(* Logix 5000 AddOnInstructionDefinition export Banner_WLS_Param_v4; software revision 33.00 *)

TYPE Banner_IOL_Port_v4 :   // UDT that has all of the data items necessary to communicate with a specific Port on a IO-Link Master
STRUCT
   Port_Controlled : INT;   // Each bit represents a port on an IO-Link Master. Set to 1 to tell AOI to control that port.
   Port_Activate : INT;   // Each bit represents a port on an IO-Link Master. When ON that port will process any commands in queue.
   Port_Read : INT;   // Each bit represents a port on an IO-Link Master. Used to determine when device AOI has requested a Read command.
   Port_Write : INT;   // Each bit represents a port on an IO-Link Master. Used to determine when device AOI has requested a Write command.
   Port_RW_Complete : INT;   // Each bit represents a port on an IO-Link Master. Tells device AOI that Read or Write request has been completed.
   Port_Device_Read : INT;
   Data_Transfer : SINT[190];   // Array to transfer data from IO-Master to device AOIs.
END_STRUCT
END_TYPE

TYPE Banner_WLS_CC_v4 :   // Tags to control color for a WLS Pro
STRUCT
   Animation : SINT;   // 0 = Off, 1 = Steady, 2 = Flash, 3 = 2 Color Flash, 4 = 2 Color Shift, 5 = Ends Steady, 6 = Ends Flash, 7 = Scroll, 8 = Center Bounce, 9 = Bounce, 10 = Center Bounce, 11 = Intensity Sweep, 12 = 2 Color Sweep, 13 = Spectrum. WLS15 Only 14 = Level Steady, 15 = Level Flash.
   Color_1 : SINT;   // 0 = Green, 1 = Red, 2 = Orange, 3 = Amber, 4 = Yellow, 5 = Lime Green, 6 = Spring Green, 7 = Cyan, 8 = Sky Blue, 9 = Blue, 10 = Violet, 11 = Magneta, 12 = Rose, 13 = Daylight White, 14 = Custom 1, 15 = Custom 2, 16 = Incandescent, 17 = Warm White, 18 = Flourescent, 19 = Neutral White, 20 = Cool White.
   Color_1_Intensity : SINT;   // 0 = High, 1 = Low, 2 = Medium, 3 = Off, 4 = Custom.
   Speed : SINT;   // 0 = Medium, 1 = Fast, 2 = Slow, 3 = Custom.
   Pulse_Pattern : SINT;   // 0 = Normal, 1 = Strobe, 2 = Three Pulse, 3 = SOS, 4 = Random.
   Color_2 : SINT;   // 0 = Green, 1 = Red, 2 = Orange, 3 = Amber, 4 = Yellow, 5 = Lime Green, 6 = Spring Green, 7 = Cyan, 8 = Sky Blue, 9 = Blue, 10 = Violet, 11 = Magneta, 12 = Rose, 13 = Daylight White, 14 = Custom 1, 15 = Custom 2, 16 = Incandescent, 17 = Warm White, 18 = Flourescent, 19 = Neutral White, 20 = Cool White.
   Color_2_Intensity : SINT;   // 0 = High, 1 = Low, 2 = Medium, 3 = Off, 4 = Custom.
   ScrollBounce : SINT;   // 0 = Solid, 1 = Blended Tail, 2 = Center Blended.
   Percent_Width_C1 : SINT;   // 1 to 100% of Color 1.
   Direction : SINT;   // 0 = Forward, 1 = Backward.
END_STRUCT
END_TYPE

TYPE Banner_WLS_DB_Config_v4 :   // Dim and Blend Mode Config.
STRUCT
   Num_of_Colors : SINT;   // 0 = 1 Color, 1 = 2 Colors, 2 = 3 colors. Number of colors to blend in variable color mode.
   Full_Scale : INT;   // 0 to 100 = Threshold Percent
   Color_1 : SINT;   // 0 = Green, 1 = Red, 2 = Orange, 3 = Amber, 4 = Yellow, 5 = Lime Green, 6 = Spring Green, 7 = Cyan, 8 = Sky Blue, 9 = Blue, 10 = Violet, 11 = Magneta, 12 = Rose, 13 = Daylight White, 14 = Custom 1, 15 = Custom 2, 16 = Incandescent, 17 = Warm White, 18 = Flourescent, 19 = Neutral White, 20 = Cool White.
   Color_1_Intensity : SINT;   // 0 = High, 1 = Low, 2 = Medium, 3 = Off, 4 = Custom
   Color_2 : SINT;   // 0 = Green, 1 = Red, 2 = Orange, 3 = Amber, 4 = Yellow, 5 = Lime Green, 6 = Spring Green, 7 = Cyan, 8 = Sky Blue, 9 = Blue, 10 = Violet, 11 = Magneta, 12 = Rose, 13 = Daylight White, 14 = Custom 1, 15 = Custom 2, 16 = Incandescent, 17 = Warm White, 18 = Flourescent, 19 = Neutral White, 20 = Cool White.
   Color_2_Intensity : SINT;   // 0 = High, 1 = Low, 2 = Medium, 3 = Off, 4 = Custom
   Color_3 : SINT;   // 0 = Green, 1 = Red, 2 = Orange, 3 = Amber, 4 = Yellow, 5 = Lime Green, 6 = Spring Green, 7 = Cyan, 8 = Sky Blue, 9 = Blue, 10 = Violet, 11 = Magneta, 12 = Rose, 13 = Daylight White, 14 = Custom 1, 15 = Custom 2, 16 = Incandescent, 17 = Warm White, 18 = Flourescent, 19 = Neutral White, 20 = Cool White.
   Color_3_Intensity : SINT;   // 0 = High, 1 = Low, 2 = Medium, 3 = Off, 4 = Custom
   Filtering : SINT;   // 0 = None, 1 = Low, 2 = Medium, 3 = High
END_STRUCT
END_TYPE

TYPE Banner_WLS_Gauge_CC_v4 :   // Parameter Data Tags for Gauge mode color control.
STRUCT
   Threshold_Enable : SINT;   // 0 = Disabled, 1 = Enabled.
   Threshold_Value_Percent : SINT;   // 0 to 100 - Threshold %
   Threshold_Comparison : SINT;   // 0 = Less than or equal to, 1 = Greater than or equal to.
   Percent_Width_of_Main_Segment : SINT;   // 0 to 100 = Percent width of color 1
   Main_CC : Banner_WLS_CC_v4;   // Color Control for the Main Lighting.
   Back_CC : Banner_WLS_CC_v4;   // Color Control for the Background Lighting.
END_STRUCT
END_TYPE

TYPE Banner_WLS_Gauge_Config_v4 :   // Tags that control Gauge Mode.
STRUCT
   Full_Scale_Value : INT;   // 0 to 100 = Threshold Percent.
   Filtering : SINT;   // 0 = None, 1 = Low, 2 = Medium, 3 = High
   Hysteresis : SINT;   // 0 = None, 1 = Low, 2 = Medium, 3 = High
   Threshold_Markers_Type : SINT;   // 0 = Off, 1= Non-Dominant, 2= Dominant.
   CC : Banner_WLS_Gauge_CC_v4[3];   // Gauge Color Control tags.
END_STRUCT
END_TYPE

TYPE Banner_WLS_Level_Config_v4 :   // Variables that Control the Level Mode of the WLS Pro.
STRUCT
   Background_Color : SINT;   // 0 = Green, 1 = Red, 2 = Orange, 3 = Amber, 4 = Yellow, 5 = Lime Green, 6 = Spring Green, 7 = Cyan, 8 = Sky Blue, 9 = Blue, 10 = Violet, 11 = Magneta, 12 = Rose, 13 = Daylight White, 14 = Custom 1, 15 = Custom 2, 16 = Incandescent, 17 = Warm White, 18 = Flourescent, 19 = Neutral White, 20 = Cool White.
   Background_Intensity : SINT;   // 0 = High, 1 = Low, 2 = Medium, 3 = Off, 4 = Custom
   Dominance : SINT;   // 0 = Non-Dominant, 1 = Dominant
   SubSegment_Style : SINT;   // 0 = Solid, 1 = Analog
   Filtering : SINT;   // 0 = None, 1 = Low, 2 = Medium, 3 = High
   Hysteresis : SINT;   // 0 = None, 1 = Low, 2 = Medium, 3 = High
   Full_Scale_Value : INT;   // Value that controls what the full scale value is
   Threshold_Marks_Type : SINT;   // WLS15 or WLF only. 0 = Off, 1 = Non-Dominant, 2 = Dominant.
   LB_Config : Banner_WLS_CC_v4;   // Level Base Configuration
   LT_Config : Banner_WLS_LT_v4[5];   // Level Threshold Configuration
END_STRUCT
END_TYPE

TYPE Banner_WLS_LT_v4 :   // Variables to configure the Level Threshold.
STRUCT
   Threshold_Enable : SINT;   // 0 = Threshold Disabled, 1 = Threshold Enabled
   Threshold_Value : SINT;   // 0 to 100 Threshold Percent
   Threshold_Comparison : SINT;   // 0 = Less than or equal to, 1 = Greater than or equal to
   Threshold_Override : SINT;   // 0 = Override not enabled, 1 = Override enabled
   Light_Control : Banner_WLS_CC_v4;   // Color Control
END_STRUCT
END_TYPE

TYPE Banner_WLS_RD_v4 :   // UDT that stores the Read Data for a WLS Pro.
STRUCT
   Master_Cycle_Time : INT;
   Min_Cycle_Time : INT;
   M_Sequence_Capability : INT;
   IO_Link_Version_ID : INT;
   Process_Data_Input_Length : INT;
   Process_Data_Output_Length : INT;
   Combined_Vendor_ID : DINT;   // IO-Link Vendor ID
   Vendor_ID1 : INT;
   Vendor_ID2 : INT;
   Combined_Device_ID : DINT;   // IO-Link Device ID
   Device_ID1 : INT;
   Device_ID2 : INT;
   Device_ID3 : INT;
   Serial_Number : STRING;
END_STRUCT
END_TYPE

TYPE Banner_WLS_Seg_Config_v4 :   // UDT for segment setup in index 66 of the parameter data.
STRUCT
   Basic_Color : SINT;   // 0 = Green, 1 = Red, 2 = Orange, 3 = Amber, 4 = Yellow, 5 = Lime Green, 6 = Spring Green, 7 = Cyan, 8 = Sky Blue, 9 = Blue, 10 = Violet, 11 = Magneta, 12 = Rose, 13 = Daylight White, 14 = Custom 1, 15 = Custom 2, 16 = Incandescent, 17 = Warm White, 18 = Flourescent, 19 = Neutral White, 20 = Cool White.
   Basic_Flash_Rate : SINT;   // 0 = Medium, 1 = Fast, 2 = Slow, 3 = Custom.
   CC : Banner_WLS_CC_v4;   // Color Control
   Manual_Segment_Offset : SINT;   // 0 to 64 = Manual Offset in LEDs.
   Manual_Segment_Width : SINT;   // 0 to 64 = Manual width in LEDs.
END_STRUCT
END_TYPE

TYPE Banner_WLS_v4 :   // All of the parameters for a WLS Pro.
STRUCT
   Initial_Global_Read : BOOL;   // Determines if all of the IO-Link data has been read into the PLC yet
   Command : INT;   // Value placed in here will activate a read or write to a specifc IO-Link Index
   Read : Banner_WLS_RD_v4;   // Read Only Data
   Write : Banner_WLS_WD_v4;   // Write Data
   Archive : Banner_WLS_WD_v4;   // Archive of the Write Data
   Reset : BOOL;   // Resets AOI. This will force a complete parameter read of the sensor.
END_STRUCT
END_TYPE

TYPE Banner_WLS_WD_v4 :   // UDT that stores the Write Data for a WLS Pro.
STRUCT
   System_Command : INT;   // See IODD file for list of commands that can be activated via the System Command interface
   Parameter_Access_Lock : SINT;   // Write access to all parameters is prohibited while value is 1. Only this parameter can be adjusted when value is 1.
   Data_Storage_Lock : SINT;   // Automatic data storage is disabled when this value is equal to 1. Read access is not affected.
   Local_Parameterization_Lock : SINT;   // Parameterization via local control elements on device is disabled.
   Local_User_Interface_Lock : SINT;   // Operation of local user interface is disabled.
   Operating_Mode_Selection : SINT;   // 0 = Segment, 1 = Run, 2 = Level, 3 = Dim & Blend, 4 = Gauge, 5 = LED
   Segment_Mode : SINT;   // 0 = Manual Segment Config. 1 trough 10 = Number of segments in Segment Mode.
   BackGround_Color : SINT;   // 0 = Green, 1 = Red, 2 = Orange, 3 = Amber, 4 = Yellow, 5 = Lime Green, 6 = Spring Green, 7 = Cyan, 8 = Sky Blue, 9 = Blue, 10 = Violet, 11 = Magneta, 12 = Rose, 13 = Daylight White, 14 = Custom 1, 15 = Custom 2, 16 = Incandescent, 17 = Warm White, 18 = Flourescent, 19 = Neutral White, 20 = Cool White.
   Background_Intensity : SINT;   // 0 = High, 1 = Low, 2 = Medium, 3 = Off, 4 = Custom
   Animation_Sync : SINT;   // 0 = Instant Update, 1 = Synchronized Update.
   SM_Config : Banner_WLS_Seg_Config_v4[11];   // Segement Mode Configuration
   LM_Config : Banner_WLS_Level_Config_v4;   // Level Mode Configuration
   Custom_Color_1_R : INT;   // 0 to 255 for Red Custom Color 1.
   Custom_Color_1_G : INT;   // 0 to 255 for Green Custom Color 1.
   Custom_Color_1_B : INT;   // 0 to 255 for Blue Custom Color 1.
   Custom_Color_2_R : INT;   // 0 to 255 for Red Custom Color 2.
   Custom_Color_2_G : INT;   // 0 to 255 for Green Custom Color 2.
   Custom_Color_2_B : INT;   // 0 to 255 for Blue Custom Color 2.
   LED_Mode_Intensity : SINT;   // 0 = High, 1 = Low, 2 = Medium, 3 = Off, 4 = Custom
   Orientation : SINT;   // 0 = Standard, 1 = Upside Down
   Custom_Intensity : SINT;   // 0 to 100 %
   Custom_Frequency : SINT;   // 0 to 255Hz
   DB_Config : Banner_WLS_DB_Config_v4;   // Dim and Blend Configuration
   G_Config : Banner_WLS_Gauge_Config_v4;   // Gauge Configuration
   Number_of_LEDs : INT;
END_STRUCT
END_TYPE

ADD_ON_INSTRUCTION Banner_WLS_Param_v4   (* revision 4.2, vendor Banner Engineering *)
// AOI to read and write parameter data to an IO-Link WLS Pro.
// Revision note:
// Updated for WLF lights.
VAR_IN_OUT
   WLS : Banner_WLS_v4; {required}
   Port_Data : Banner_IOL_Port_v4; {required}
END_VAR
VAR_INPUT
   Port : INT; {required}   // Port Number that device is plugged into.
   Type : SINT; {required}   // 0 = WLS27, 1 = WLS15, 2 = WLF
END_VAR
VAR
   Local_Control : DINT; {access None}
   Global_Read_Command_Value : INT; {access None}
   Global_Write_Command_Value : INT; {access None}
   Command_Being_Processed : BOOL; {access None}
   Update_Archive : BOOL; {access None}
   Index_Write_Inprocess : DINT; {access None}
   Index_Write_Control : DINT; {access None}
   Inprocess_Index : DINT; {access None}
   IndexR : DINT; {access None}   // Index keeping track of Reads in an array.
   S_Index : DINT; {access None}
   IndexW : DINT; {access None}   // Index keeping track of Writes in an array.
   SW_Index : DINT; {access None}
   Index_Segment_Read : DINT; {access None}
   LT_Index : DINT; {access None}
   IndexW2 : DINT; {access None}
   LTW_Index : DINT; {access None}
   G_Index : DINT; {access None}
   IndexW3 : DINT; {access None}
   GW_Index : DINT; {access None}
END_VAR

ROUTINE Logic   (* ladder *)
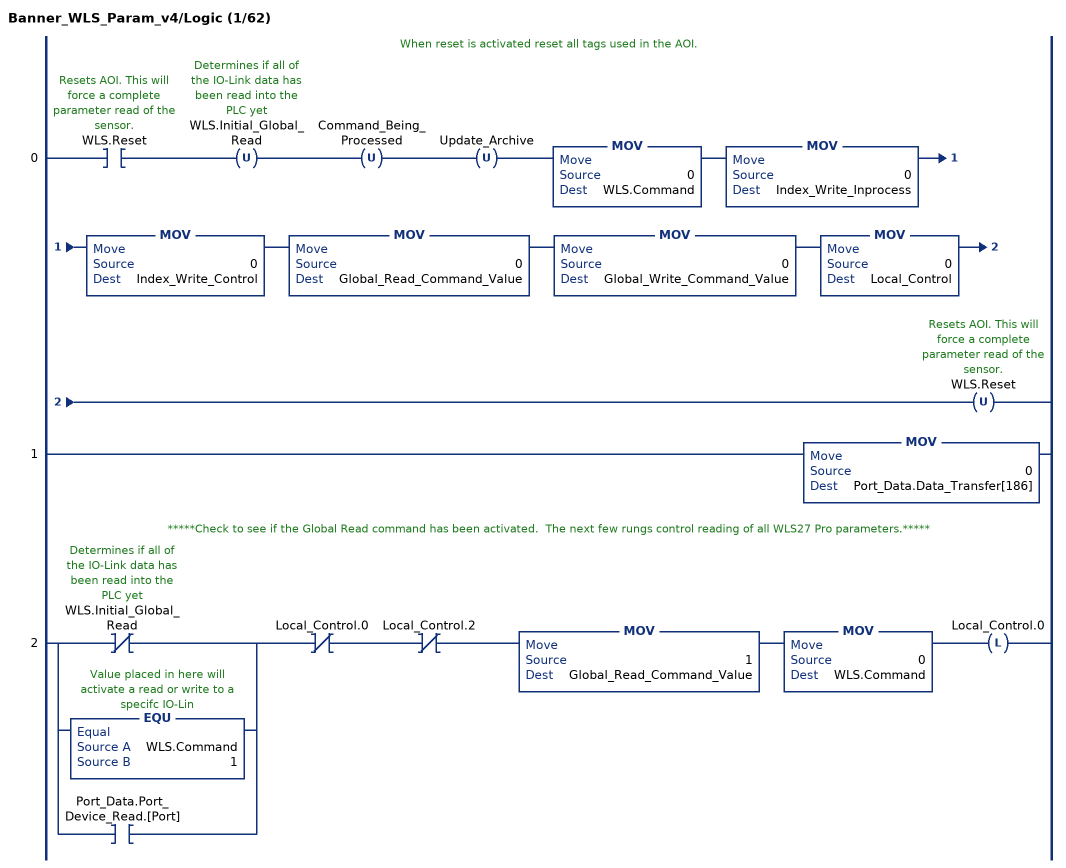
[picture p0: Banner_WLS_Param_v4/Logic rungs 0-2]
   // When reset is activated reset all tags used in the AOI.
   0: XIC(WLS.Reset)OTU(WLS.Initial_Global_Read)OTU(Command_Being_Processed)OTU(Update_Archive)MOV(0,WLS.Command)MOV(0,Index_Write_Inprocess)MOV(0,Index_Write_Control)MOV(0,Global_Read_Command_Value)MOV(0,Global_Write_Command_Value)MOV(0,Local_Control)OTU(WLS.Reset);
   1: MOV(0,Port_Data.Data_Transfer[186]);
   // *****Check to see if the Global Read command has been activated.  The next few rungs control reading of all WLS27 Pro parameters.*****
   2: [XIO(WLS.Initial_Global_Read) ,EQU(WLS.Command,1) ,XIC(Port_Data.Port_Device_Read.[Port]) ]XIO(Local_Control.0)XIO(Local_Control.2)MOV(1,Global_Read_Command_Value)MOV(0,WLS.Command)OTL(Local_Control.0);
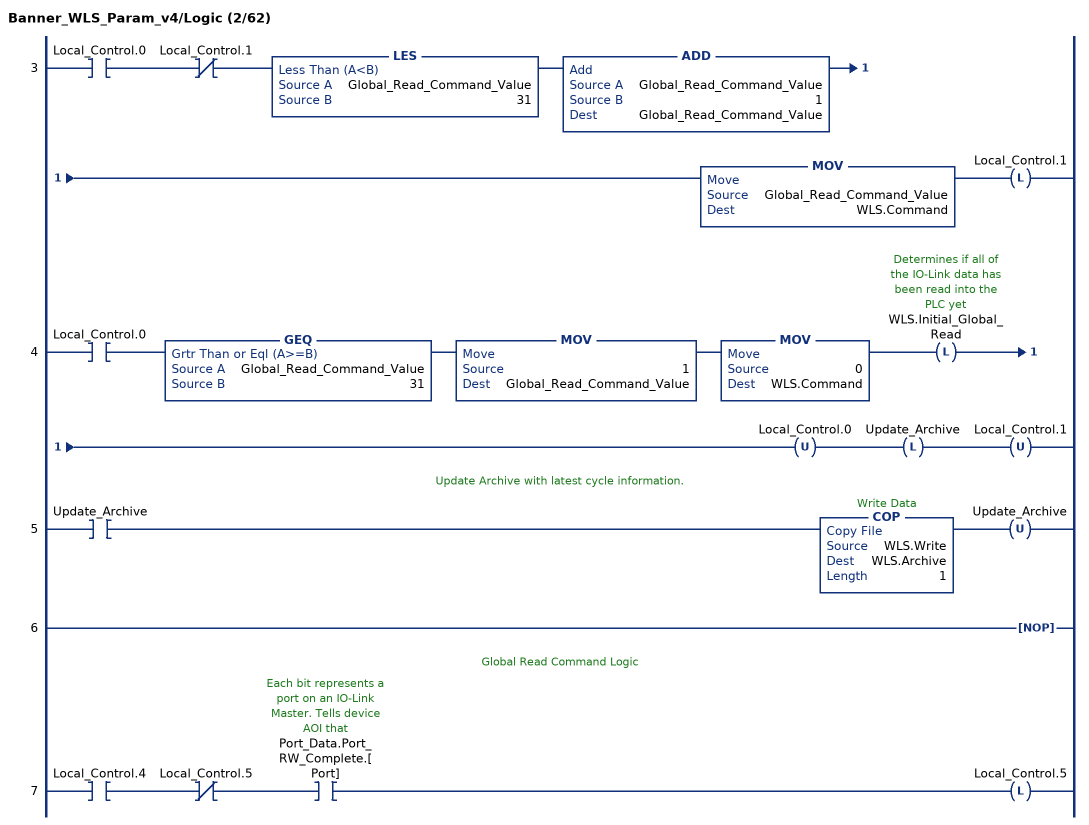
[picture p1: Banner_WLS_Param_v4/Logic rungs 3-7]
   3: XIC(Local_Control.0)XIO(Local_Control.1)LES(Global_Read_Command_Value,31)ADD(Global_Read_Command_Value,1,Global_Read_Command_Value)MOV(Global_Read_Command_Value,WLS.Command)OTL(Local_Control.1);
   4: XIC(Local_Control.0)GEQ(Global_Read_Command_Value,31)MOV(1,Global_Read_Command_Value)MOV(0,WLS.Command)OTL(WLS.Initial_Global_Read)OTU(Local_Control.0)OTL(Update_Archive)OTU(Local_Control.1);
   // Update Archive with latest cycle information.
   5: XIC(Update_Archive)COP(WLS.Write,WLS.Archive,1)OTU(Update_Archive);
   6: NOP();
   // Global Read Command Logic
   7: XIC(Local_Control.4)XIO(Local_Control.5)XIC(Port_Data.Port_RW_Complete.[Port])OTL(Local_Control.5);
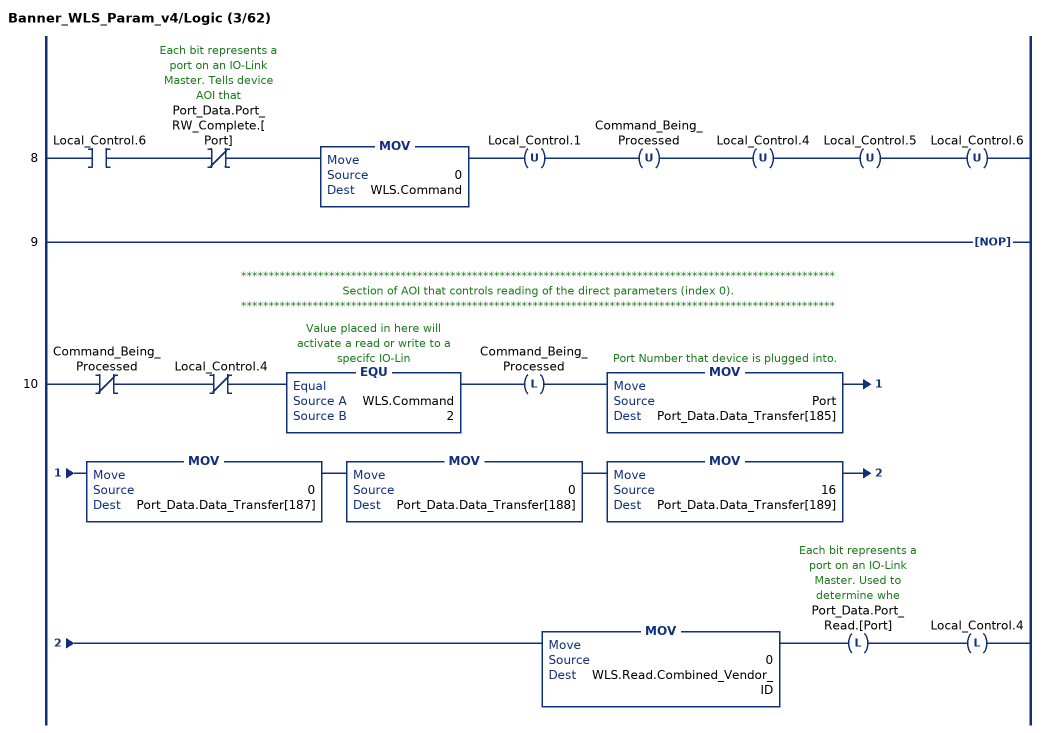
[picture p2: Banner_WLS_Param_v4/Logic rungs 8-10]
   8: XIC(Local_Control.6)XIO(Port_Data.Port_RW_Complete.[Port])MOV(0,WLS.Command)OTU(Local_Control.1)OTU(Command_Being_Processed)OTU(Local_Control.4)OTU(Local_Control.5)OTU(Local_Control.6);
   9: NOP();
   // ************************************************************************************************************
   // Section of AOI that controls reading of the direct parameters (index 0).
   // ************************************************************************************************************
   10: XIO(Command_Being_Processed)XIO(Local_Control.4)EQU(WLS.Command,2)OTL(Command_Being_Processed)MOV(Port,Port_Data.Data_Transfer[185])MOV(0,Port_Data.Data_Transfer[187])MOV(0,Port_Data.Data_Transfer[188])MOV(16,Port_Data.Data_Transfer[189])MOV(0,WLS.Read.Combined_Vendor_ID)OTL(Port_Data.Port_Read.[Port])OTL(Local_Control.4);
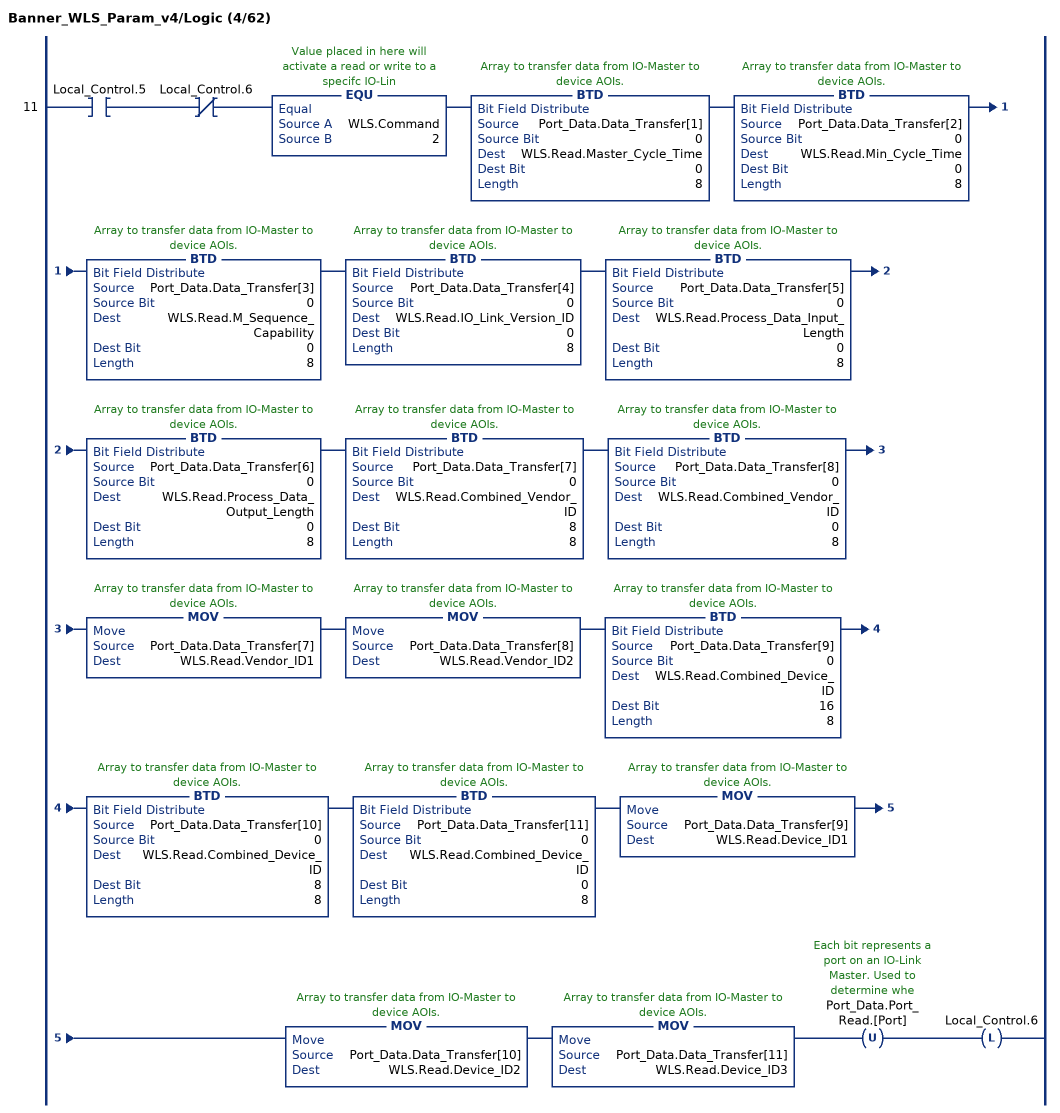
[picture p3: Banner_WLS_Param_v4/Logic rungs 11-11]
   11: XIC(Local_Control.5)XIO(Local_Control.6)EQU(WLS.Command,2)BTD(Port_Data.Data_Transfer[1],0,WLS.Read.Master_Cycle_Time,0,8)BTD(Port_Data.Data_Transfer[2],0,WLS.Read.Min_Cycle_Time,0,8)BTD(Port_Data.Data_Transfer[3],0,WLS.Read.M_Sequence_Capability,0,8)BTD(Port_Data.Data_Transfer[4],0,WLS.Read.IO_Link_Version_ID,0,8)BTD(Port_Data.Data_Transfer[5],0,WLS.Read.Process_Data_Input_Length,0,8)BTD(Port_Data.Data_Transfer[6],0,WLS.Read.Process_Data_Output_Length,0,8)BTD(Port_Data.Data_Transfer[7],0,WLS.Read.Combined_Vendor_ID,8,8)BTD(Port_Data.Data_Transfer[8],0,WLS.Read.Combined_Vendor_ID,0,8)MOV(Port_Data.Data_Transfer[7],WLS.Read.Vendor_ID1)MOV(Port_Data.Data_Transfer[8],WLS.Read.Vendor_ID2)BTD(Port_Data.Data_Transfer[9],0,WLS.Read.Combined_Device_ID,16,8)BTD(Port_Data.Data_Transfer[10],0,WLS.Read.Combined_Device_ID,8,8)BTD(Port_Data.Data_Transfer[11],0,WLS.Read.Combined_Device_ID,0,8)MOV(Port_Data.Data_Transfer[9],WLS.Read.Device_ID1)MOV(Port_Data.Data_Transfer[10],WLS.Read.Device_ID2)MOV(Port_Data.Data_Transfer[11],WLS.Read.Device_ID3)OTU(Port_Data.Port_Read.[Port])OTL(Local_Control.6);
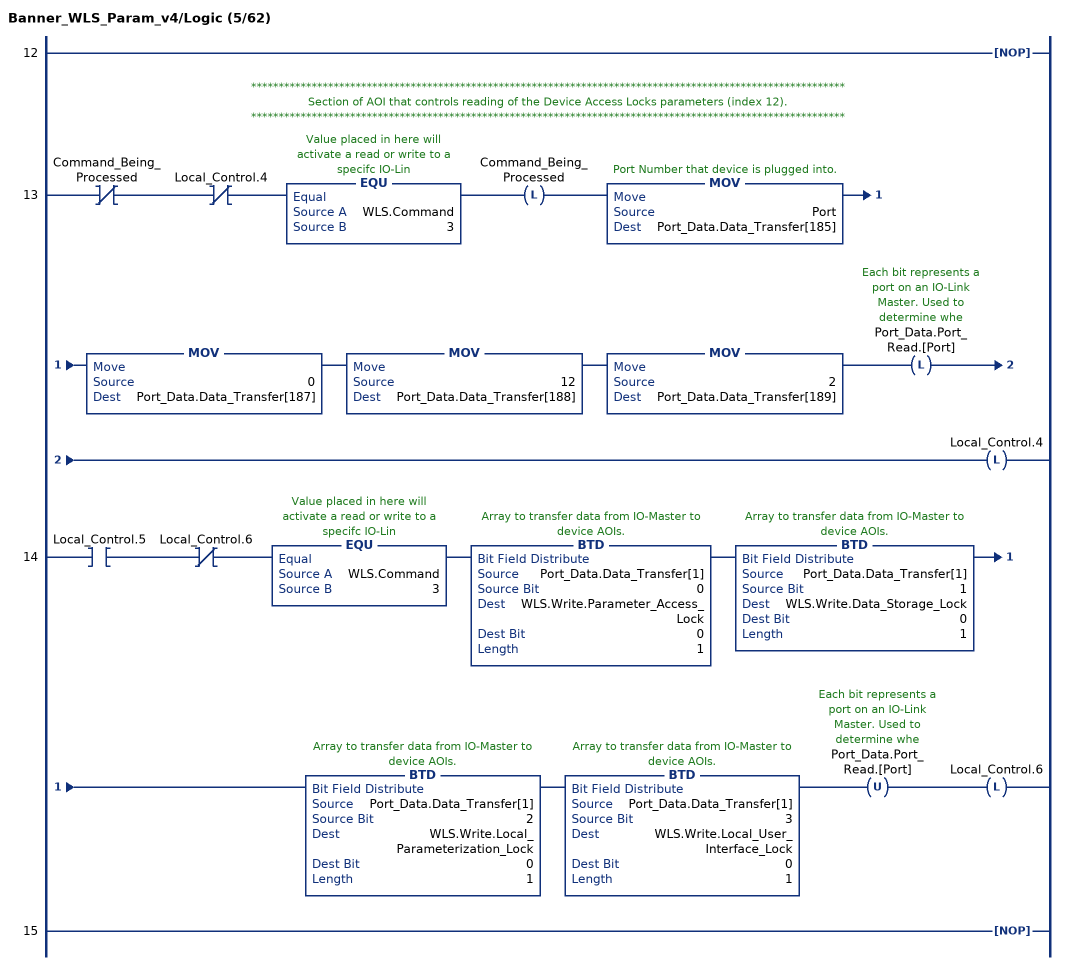
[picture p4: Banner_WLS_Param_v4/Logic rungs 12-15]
   12: NOP();
   // ************************************************************************************************************
   // Section of AOI that controls reading of the Device Access Locks parameters (index 12).
   // ************************************************************************************************************
   13: XIO(Command_Being_Processed)XIO(Local_Control.4)EQU(WLS.Command,3)OTL(Command_Being_Processed)MOV(Port,Port_Data.Data_Transfer[185])MOV(0,Port_Data.Data_Transfer[187])MOV(12,Port_Data.Data_Transfer[188])MOV(2,Port_Data.Data_Transfer[189])OTL(Port_Data.Port_Read.[Port])OTL(Local_Control.4);
   14: XIC(Local_Control.5)XIO(Local_Control.6)EQU(WLS.Command,3)BTD(Port_Data.Data_Transfer[1],0,WLS.Write.Parameter_Access_Lock,0,1)BTD(Port_Data.Data_Transfer[1],1,WLS.Write.Data_Storage_Lock,0,1)BTD(Port_Data.Data_Transfer[1],2,WLS.Write.Local_Parameterization_Lock,0,1)BTD(Port_Data.Data_Transfer[1],3,WLS.Write.Local_User_Interface_Lock,0,1)OTU(Port_Data.Port_Read.[Port])OTL(Local_Control.6);
   15: NOP();
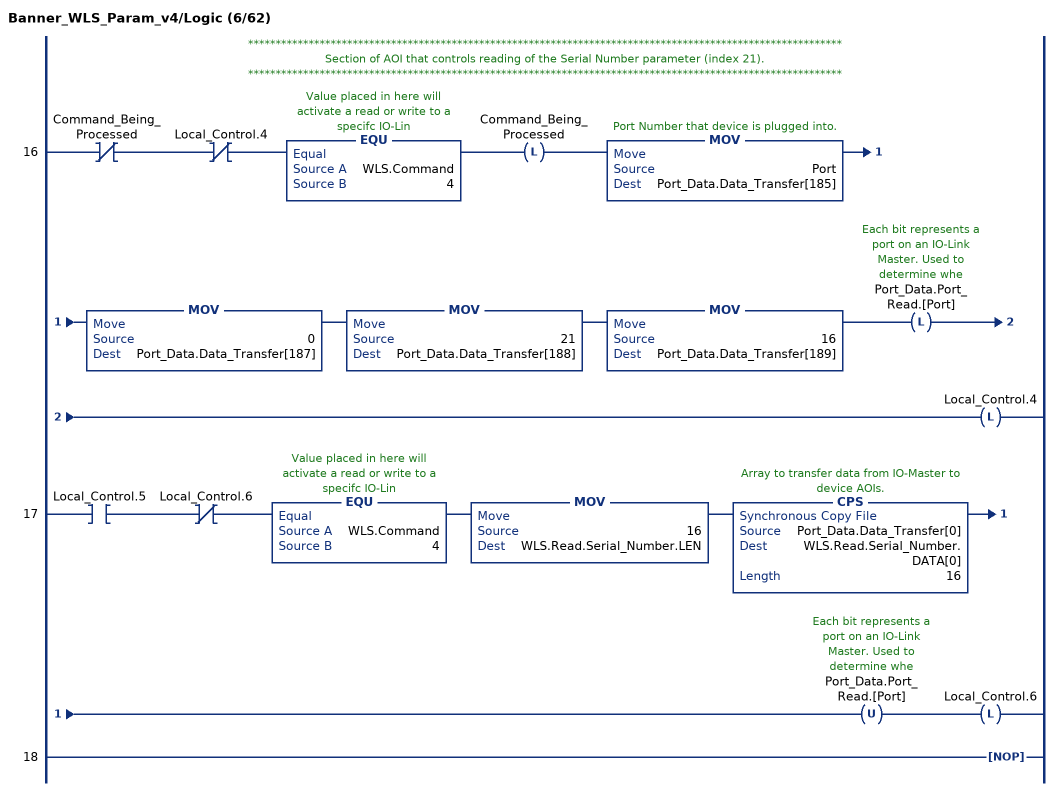
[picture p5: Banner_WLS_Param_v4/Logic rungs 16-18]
   // ************************************************************************************************************
   // Section of AOI that controls reading of the Serial Number parameter (index 21).
   // ************************************************************************************************************
   16: XIO(Command_Being_Processed)XIO(Local_Control.4)EQU(WLS.Command,4)OTL(Command_Being_Processed)MOV(Port,Port_Data.Data_Transfer[185])MOV(0,Port_Data.Data_Transfer[187])MOV(21,Port_Data.Data_Transfer[188])MOV(16,Port_Data.Data_Transfer[189])OTL(Port_Data.Port_Read.[Port])OTL(Local_Control.4);
   17: XIC(Local_Control.5)XIO(Local_Control.6)EQU(WLS.Command,4)MOV(16,WLS.Read.Serial_Number.LEN)CPS(Port_Data.Data_Transfer[0],WLS.Read.Serial_Number.DATA[0],16)OTU(Port_Data.Port_Read.[Port])OTL(Local_Control.6);
   18: NOP();
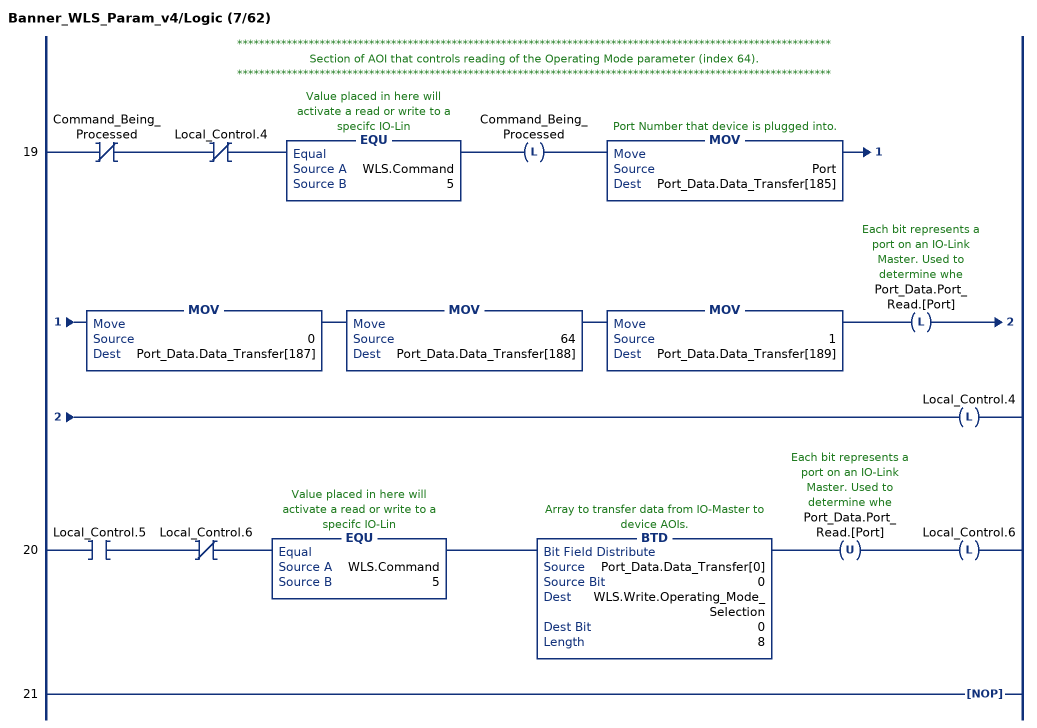
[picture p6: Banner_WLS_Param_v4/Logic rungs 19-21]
   // ************************************************************************************************************
   // Section of AOI that controls reading of the Operating Mode parameter (index 64).
   // ************************************************************************************************************
   19: XIO(Command_Being_Processed)XIO(Local_Control.4)EQU(WLS.Command,5)OTL(Command_Being_Processed)MOV(Port,Port_Data.Data_Transfer[185])MOV(0,Port_Data.Data_Transfer[187])MOV(64,Port_Data.Data_Transfer[188])MOV(1,Port_Data.Data_Transfer[189])OTL(Port_Data.Port_Read.[Port])OTL(Local_Control.4);
   20: XIC(Local_Control.5)XIO(Local_Control.6)EQU(WLS.Command,5)BTD(Port_Data.Data_Transfer[0],0,WLS.Write.Operating_Mode_Selection,0,8)OTU(Port_Data.Port_Read.[Port])OTL(Local_Control.6);
   21: NOP();
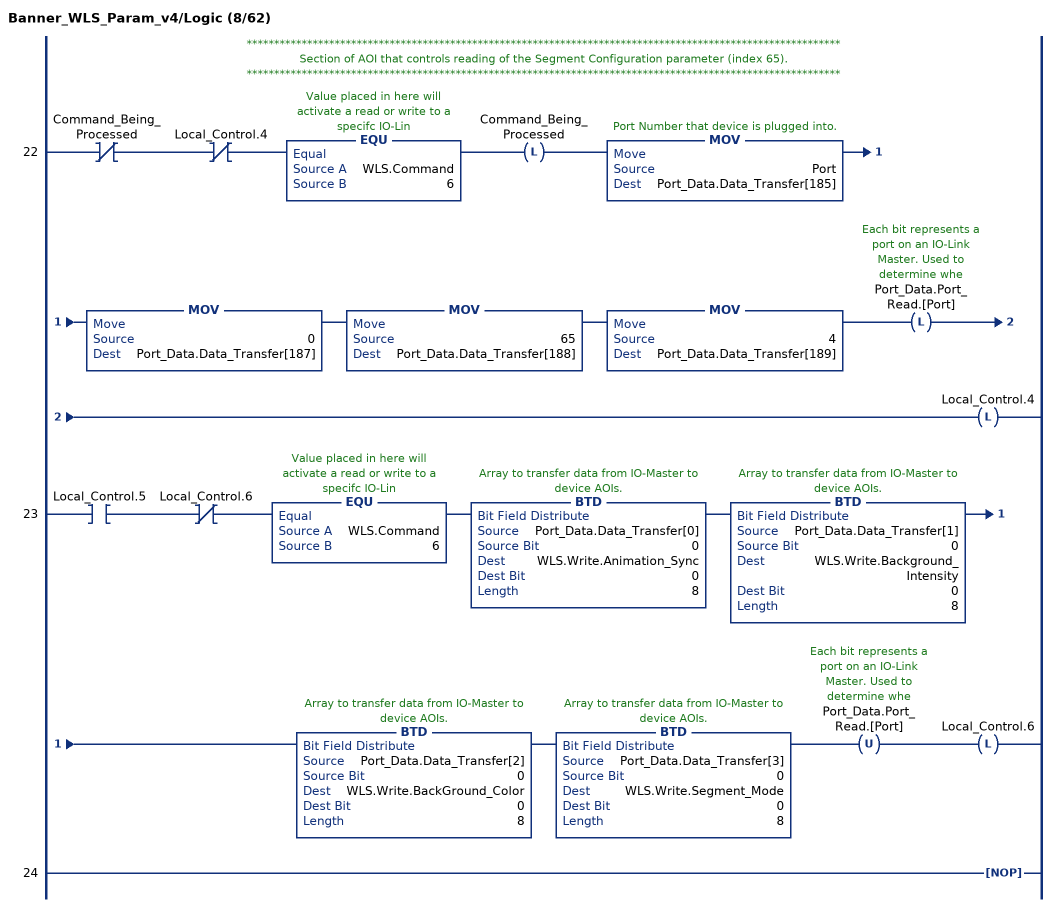
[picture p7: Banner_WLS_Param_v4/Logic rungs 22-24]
   // ************************************************************************************************************
   // Section of AOI that controls reading of the Segment Configuration parameter (index 65).
   // ************************************************************************************************************
   22: XIO(Command_Being_Processed)XIO(Local_Control.4)EQU(WLS.Command,6)OTL(Command_Being_Processed)MOV(Port,Port_Data.Data_Transfer[185])MOV(0,Port_Data.Data_Transfer[187])MOV(65,Port_Data.Data_Transfer[188])MOV(4,Port_Data.Data_Transfer[189])OTL(Port_Data.Port_Read.[Port])OTL(Local_Control.4);
   23: XIC(Local_Control.5)XIO(Local_Control.6)EQU(WLS.Command,6)BTD(Port_Data.Data_Transfer[0],0,WLS.Write.Animation_Sync,0,8)BTD(Port_Data.Data_Transfer[1],0,WLS.Write.Background_Intensity,0,8)BTD(Port_Data.Data_Transfer[2],0,WLS.Write.BackGround_Color,0,8)BTD(Port_Data.Data_Transfer[3],0,WLS.Write.Segment_Mode,0,8)OTU(Port_Data.Port_Read.[Port])OTL(Local_Control.6);
   24: NOP();
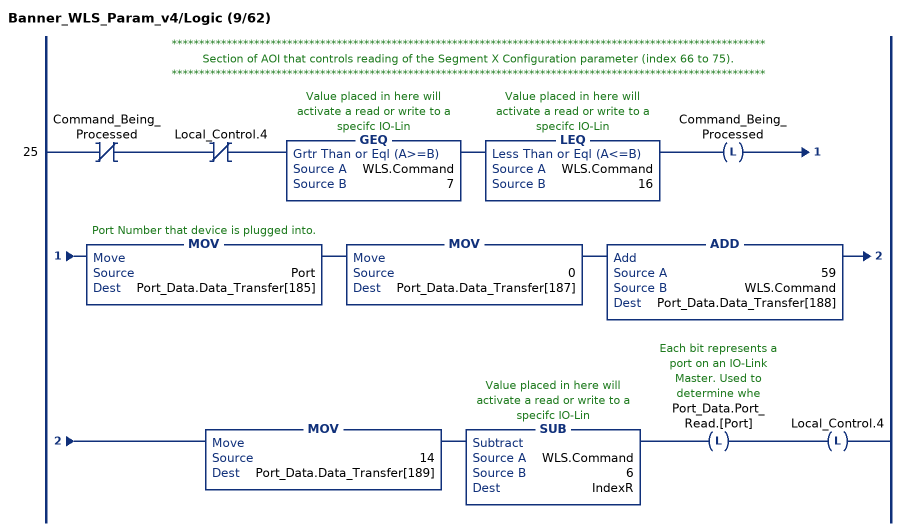
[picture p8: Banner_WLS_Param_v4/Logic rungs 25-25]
   // ************************************************************************************************************
   // Section of AOI that controls reading of the Segment X Configuration parameter (index 66 to 75).
   // ************************************************************************************************************
   25: XIO(Command_Being_Processed)XIO(Local_Control.4)GEQ(WLS.Command,7)LEQ(WLS.Command,16)OTL(Command_Being_Processed)MOV(Port,Port_Data.Data_Transfer[185])MOV(0,Port_Data.Data_Transfer[187])ADD(59,WLS.Command,Port_Data.Data_Transfer[188])MOV(14,Port_Data.Data_Transfer[189])SUB(WLS.Command,6,IndexR)OTL(Port_Data.Port_Read.[Port])OTL(Local_Control.4);
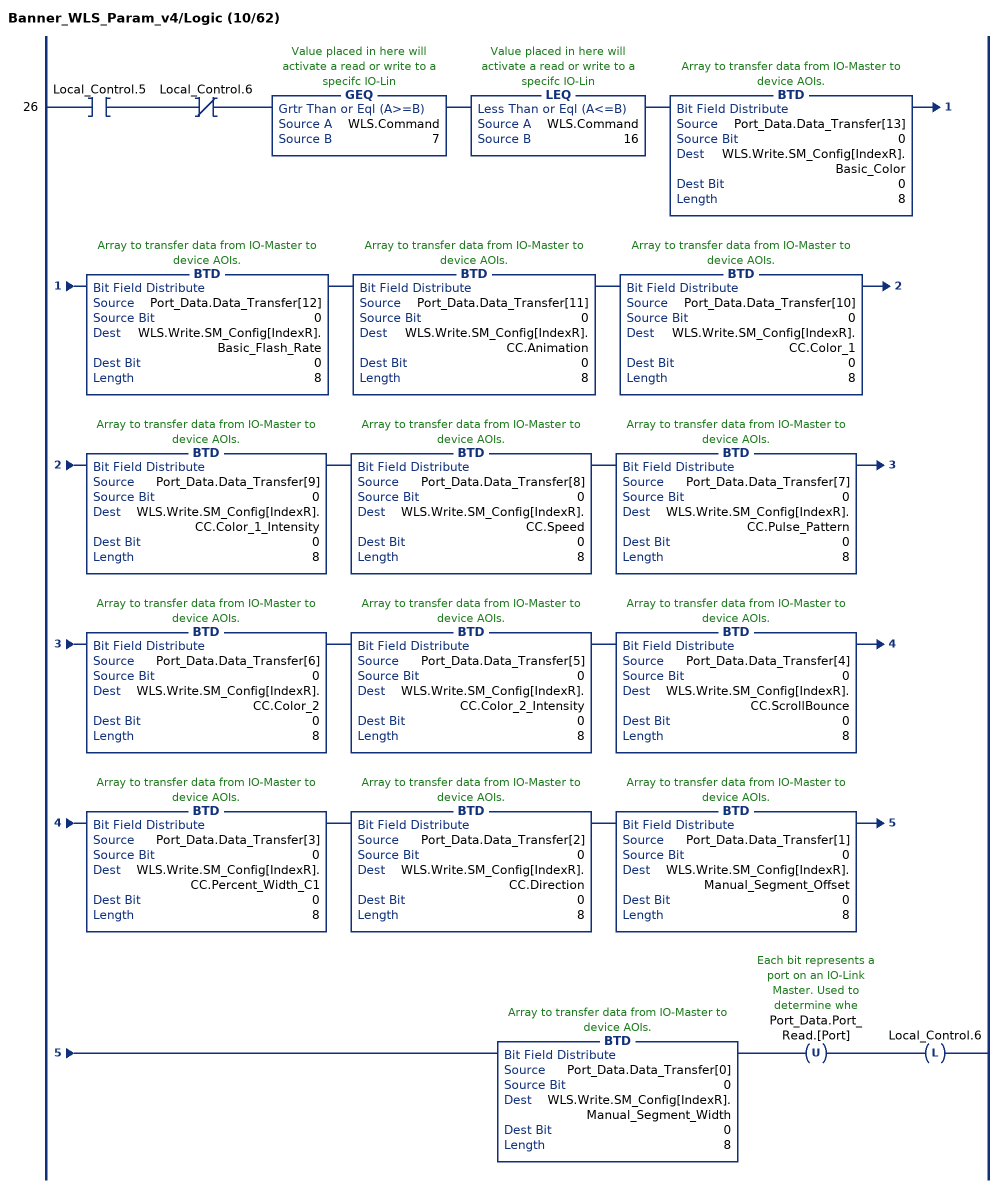
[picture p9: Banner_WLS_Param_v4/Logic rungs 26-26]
   26: XIC(Local_Control.5)XIO(Local_Control.6)GEQ(WLS.Command,7)LEQ(WLS.Command,16)BTD(Port_Data.Data_Transfer[13],0,WLS.Write.SM_Config[IndexR].Basic_Color,0,8)BTD(Port_Data.Data_Transfer[12],0,WLS.Write.SM_Config[IndexR].Basic_Flash_Rate,0,8)BTD(Port_Data.Data_Transfer[11],0,WLS.Write.SM_Config[IndexR].CC.Animation,0,8)BTD(Port_Data.Data_Transfer[10],0,WLS.Write.SM_Config[IndexR].CC.Color_1,0,8)BTD(Port_Data.Data_Transfer[9],0,WLS.Write.SM_Config[IndexR].CC.Color_1_Intensity,0,8)BTD(Port_Data.Data_Transfer[8],0,WLS.Write.SM_Config[IndexR].CC.Speed,0,8)BTD(Port_Data.Data_Transfer[7],0,WLS.Write.SM_Config[IndexR].CC.Pulse_Pattern,0,8)BTD(Port_Data.Data_Transfer[6],0,WLS.Write.SM_Config[IndexR].CC.Color_2,0,8)BTD(Port_Data.Data_Transfer[5],0,WLS.Write.SM_Config[IndexR].CC.Color_2_Intensity,0,8)BTD(Port_Data.Data_Transfer[4],0,WLS.Write.SM_Config[IndexR].CC.ScrollBounce,0,8)BTD(Port_Data.Data_Transfer[3],0,WLS.Write.SM_Config[IndexR].CC.Percent_Width_C1,0,8)BTD(Port_Data.Data_Transfer[2],0,WLS.Write.SM_Config[IndexR].CC.Direction,0,8)BTD(Port_Data.Data_Transfer[1],0,WLS.Write.SM_Config[IndexR].Manual_Segment_Offset,0,8)BTD(Port_Data.Data_Transfer[0],0,WLS.Write.SM_Config[IndexR].Manual_Segment_Width,0,8)OTU(Port_Data.Port_Read.[Port])OTL(Local_Control.6);
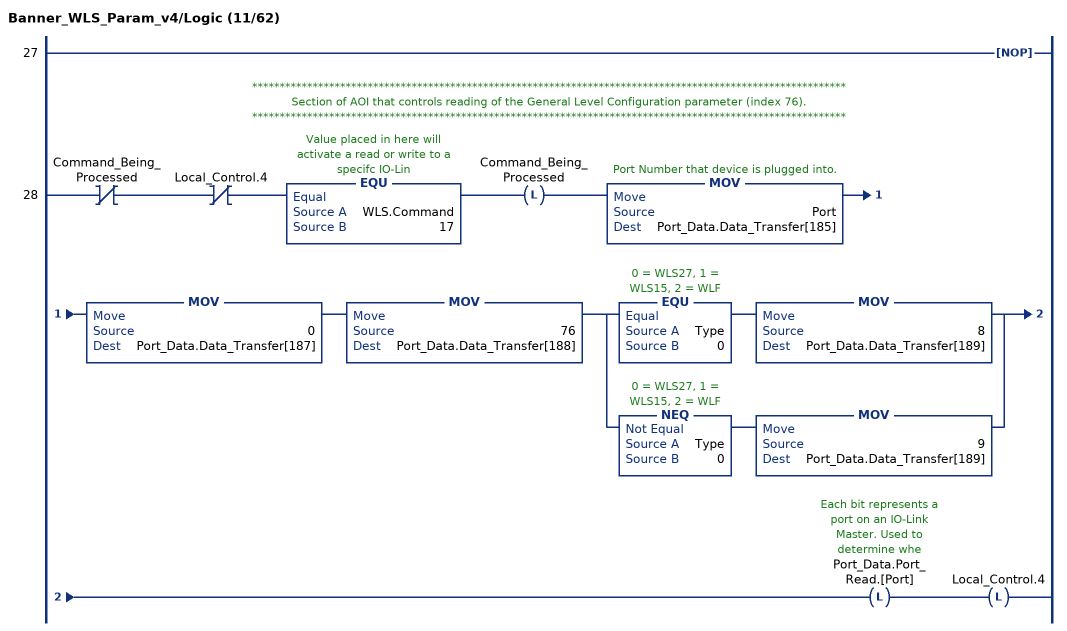
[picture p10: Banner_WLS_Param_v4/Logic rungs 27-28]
   27: NOP();
   // ************************************************************************************************************
   // Section of AOI that controls reading of the General Level Configuration parameter (index 76).
   // ************************************************************************************************************
   28: XIO(Command_Being_Processed)XIO(Local_Control.4)EQU(WLS.Command,17)OTL(Command_Being_Processed)MOV(Port,Port_Data.Data_Transfer[185])MOV(0,Port_Data.Data_Transfer[187])MOV(76,Port_Data.Data_Transfer[188])[EQU(Type,0) MOV(8,Port_Data.Data_Transfer[189]) ,NEQ(Type,0) MOV(9,Port_Data.Data_Transfer[189]) ]OTL(Port_Data.Port_Read.[Port])OTL(Local_Control.4);
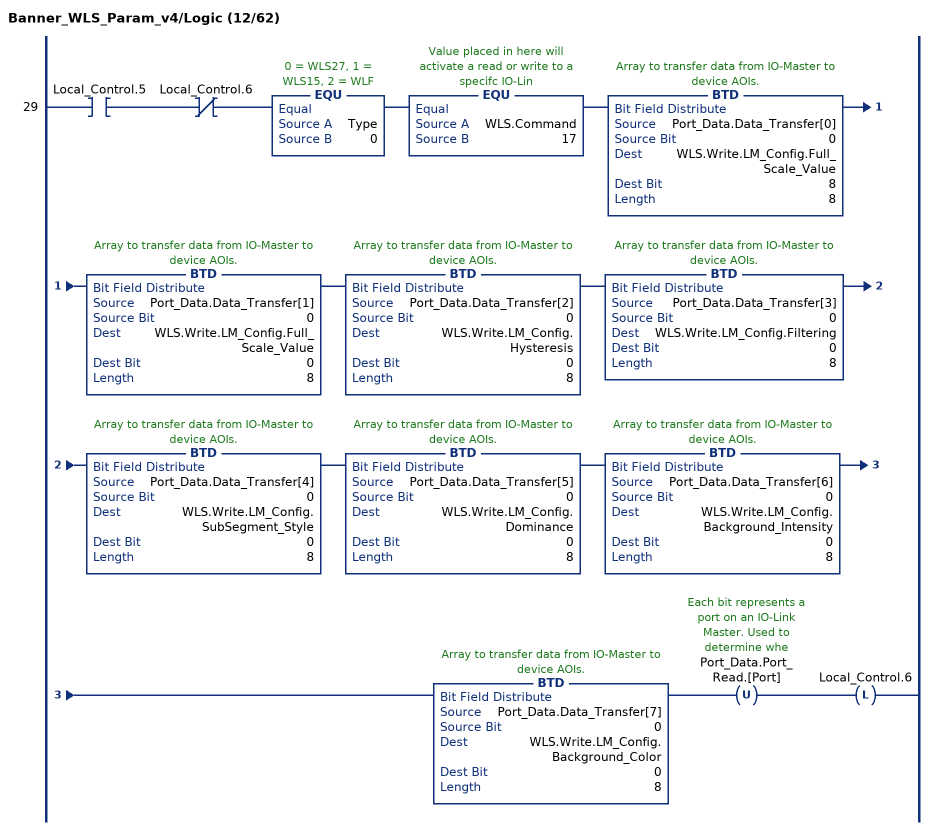
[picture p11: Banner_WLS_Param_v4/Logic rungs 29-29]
   29: XIC(Local_Control.5)XIO(Local_Control.6)EQU(Type,0)EQU(WLS.Command,17)BTD(Port_Data.Data_Transfer[0],0,WLS.Write.LM_Config.Full_Scale_Value,8,8)BTD(Port_Data.Data_Transfer[1],0,WLS.Write.LM_Config.Full_Scale_Value,0,8)BTD(Port_Data.Data_Transfer[2],0,WLS.Write.LM_Config.Hysteresis,0,8)BTD(Port_Data.Data_Transfer[3],0,WLS.Write.LM_Config.Filtering,0,8)BTD(Port_Data.Data_Transfer[4],0,WLS.Write.LM_Config.SubSegment_Style,0,8)BTD(Port_Data.Data_Transfer[5],0,WLS.Write.LM_Config.Dominance,0,8)BTD(Port_Data.Data_Transfer[6],0,WLS.Write.LM_Config.Background_Intensity,0,8)BTD(Port_Data.Data_Transfer[7],0,WLS.Write.LM_Config.Background_Color,0,8)OTU(Port_Data.Port_Read.[Port])OTL(Local_Control.6);
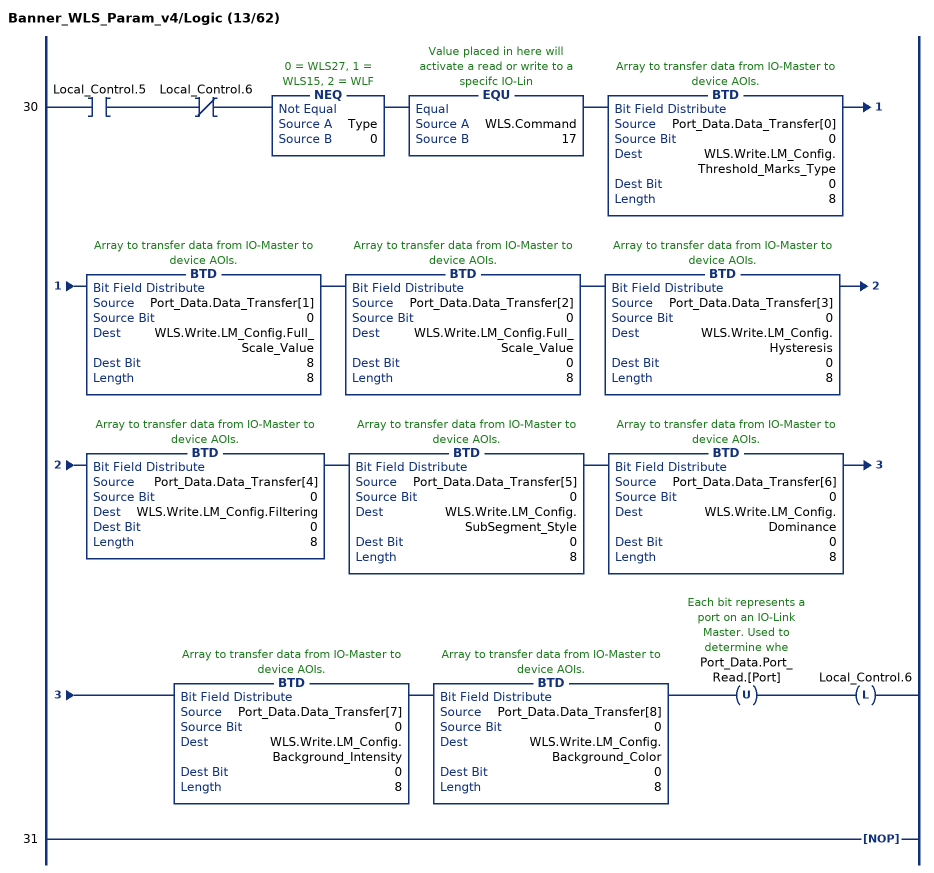
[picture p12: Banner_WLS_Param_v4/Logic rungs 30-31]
   30: XIC(Local_Control.5)XIO(Local_Control.6)NEQ(Type,0)EQU(WLS.Command,17)BTD(Port_Data.Data_Transfer[0],0,WLS.Write.LM_Config.Threshold_Marks_Type,0,8)BTD(Port_Data.Data_Transfer[1],0,WLS.Write.LM_Config.Full_Scale_Value,8,8)BTD(Port_Data.Data_Transfer[2],0,WLS.Write.LM_Config.Full_Scale_Value,0,8)BTD(Port_Data.Data_Transfer[3],0,WLS.Write.LM_Config.Hysteresis,0,8)BTD(Port_Data.Data_Transfer[4],0,WLS.Write.LM_Config.Filtering,0,8)BTD(Port_Data.Data_Transfer[5],0,WLS.Write.LM_Config.SubSegment_Style,0,8)BTD(Port_Data.Data_Transfer[6],0,WLS.Write.LM_Config.Dominance,0,8)BTD(Port_Data.Data_Transfer[7],0,WLS.Write.LM_Config.Background_Intensity,0,8)BTD(Port_Data.Data_Transfer[8],0,WLS.Write.LM_Config.Background_Color,0,8)OTU(Port_Data.Port_Read.[Port])OTL(Local_Control.6);
   31: NOP();
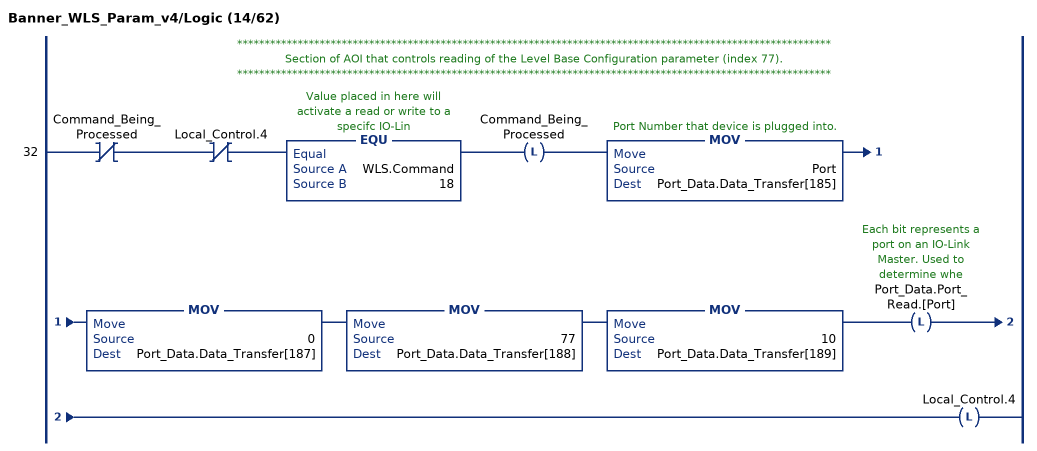
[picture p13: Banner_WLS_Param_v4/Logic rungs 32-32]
   // ************************************************************************************************************
   // Section of AOI that controls reading of the Level Base Configuration parameter (index 77).
   // ************************************************************************************************************
   32: XIO(Command_Being_Processed)XIO(Local_Control.4)EQU(WLS.Command,18)OTL(Command_Being_Processed)MOV(Port,Port_Data.Data_Transfer[185])MOV(0,Port_Data.Data_Transfer[187])MOV(77,Port_Data.Data_Transfer[188])MOV(10,Port_Data.Data_Transfer[189])OTL(Port_Data.Port_Read.[Port])OTL(Local_Control.4);
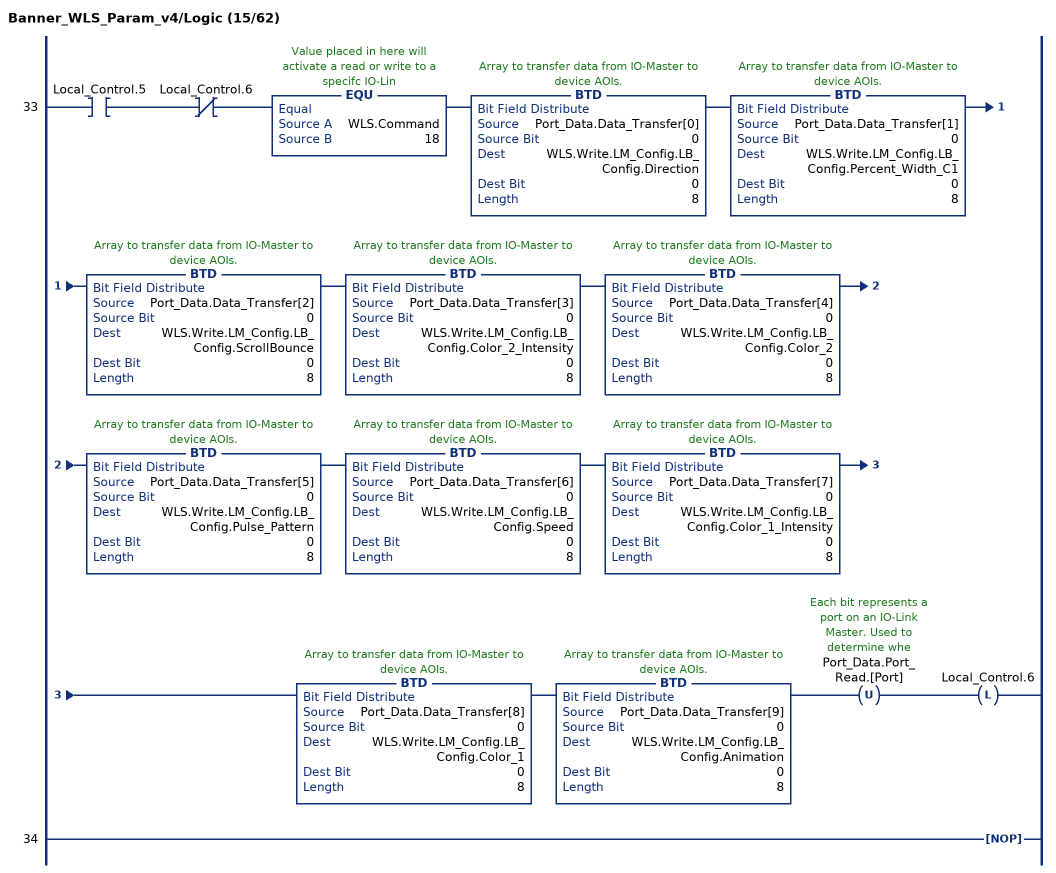
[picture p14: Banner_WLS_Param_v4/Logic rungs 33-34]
   33: XIC(Local_Control.5)XIO(Local_Control.6)EQU(WLS.Command,18)BTD(Port_Data.Data_Transfer[0],0,WLS.Write.LM_Config.LB_Config.Direction,0,8)BTD(Port_Data.Data_Transfer[1],0,WLS.Write.LM_Config.LB_Config.Percent_Width_C1,0,8)BTD(Port_Data.Data_Transfer[2],0,WLS.Write.LM_Config.LB_Config.ScrollBounce,0,8)BTD(Port_Data.Data_Transfer[3],0,WLS.Write.LM_Config.LB_Config.Color_2_Intensity,0,8)BTD(Port_Data.Data_Transfer[4],0,WLS.Write.LM_Config.LB_Config.Color_2,0,8)BTD(Port_Data.Data_Transfer[5],0,WLS.Write.LM_Config.LB_Config.Pulse_Pattern,0,8)BTD(Port_Data.Data_Transfer[6],0,WLS.Write.LM_Config.LB_Config.Speed,0,8)BTD(Port_Data.Data_Transfer[7],0,WLS.Write.LM_Config.LB_Config.Color_1_Intensity,0,8)BTD(Port_Data.Data_Transfer[8],0,WLS.Write.LM_Config.LB_Config.Color_1,0,8)BTD(Port_Data.Data_Transfer[9],0,WLS.Write.LM_Config.LB_Config.Animation,0,8)OTU(Port_Data.Port_Read.[Port])OTL(Local_Control.6);
   34: NOP();
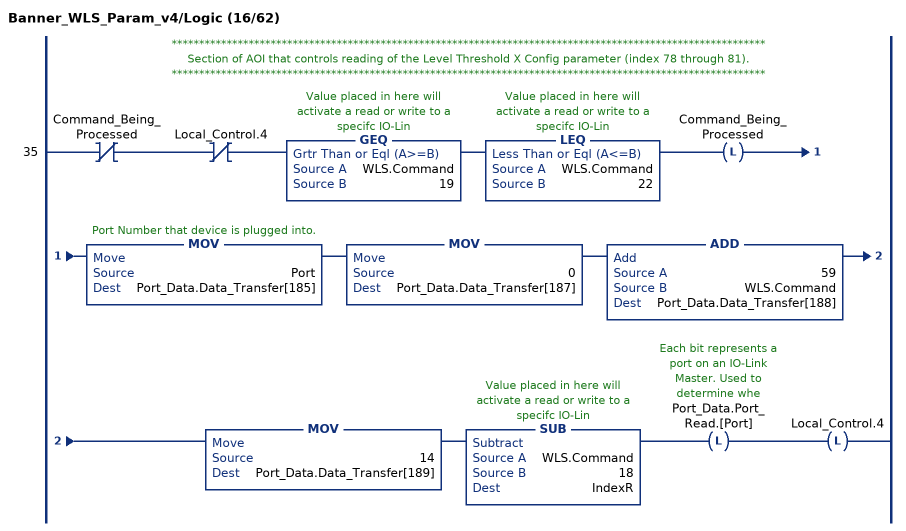
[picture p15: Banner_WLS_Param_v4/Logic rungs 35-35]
   // ************************************************************************************************************
   // Section of AOI that controls reading of the Level Threshold X Config parameter (index 78 through 81).
   // ************************************************************************************************************
   35: XIO(Command_Being_Processed)XIO(Local_Control.4)GEQ(WLS.Command,19)LEQ(WLS.Command,22)OTL(Command_Being_Processed)MOV(Port,Port_Data.Data_Transfer[185])MOV(0,Port_Data.Data_Transfer[187])ADD(59,WLS.Command,Port_Data.Data_Transfer[188])MOV(14,Port_Data.Data_Transfer[189])SUB(WLS.Command,18,IndexR)OTL(Port_Data.Port_Read.[Port])OTL(Local_Control.4);
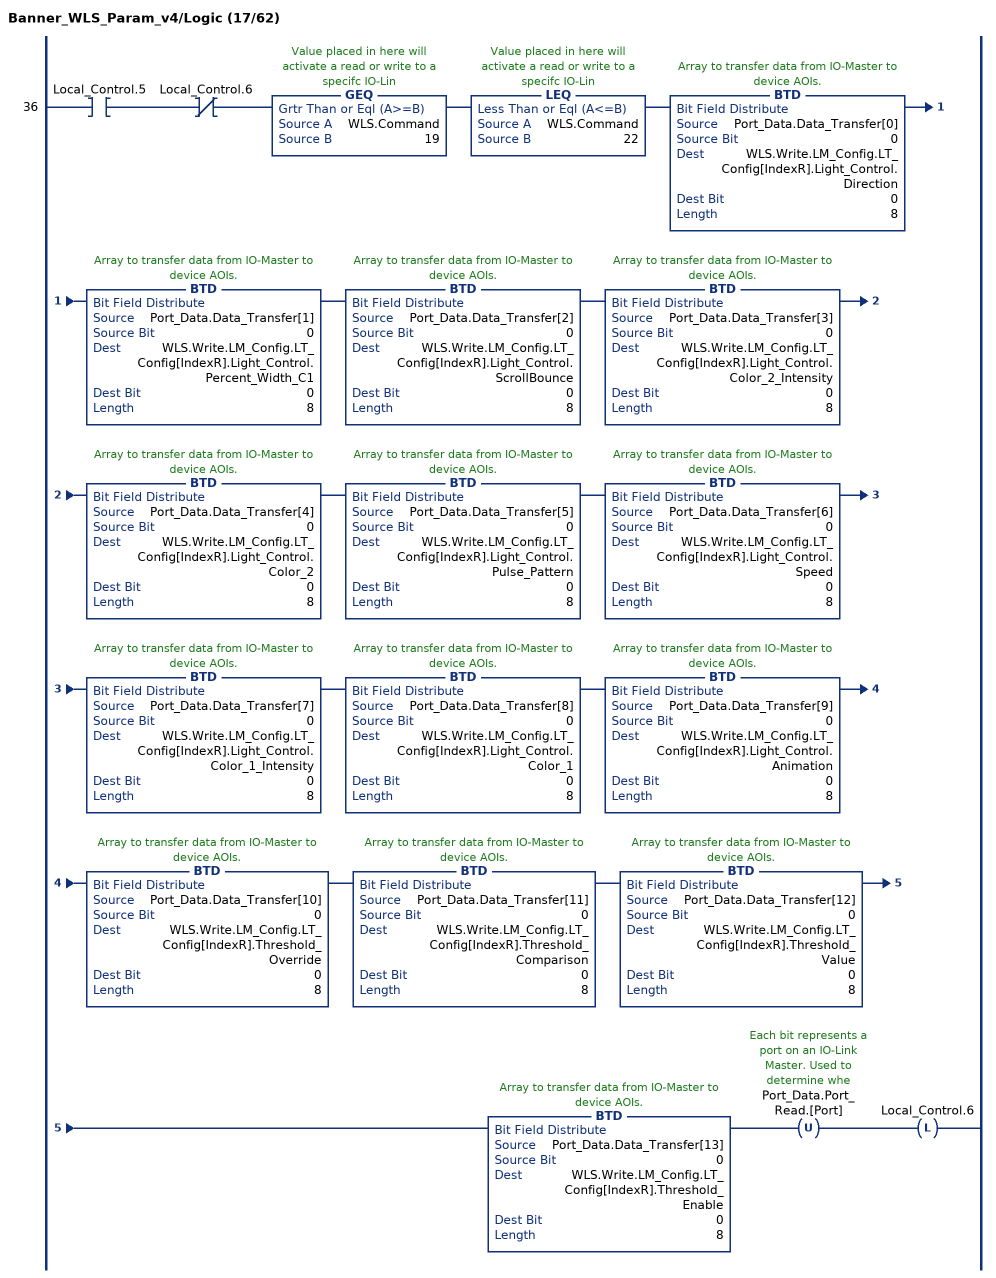
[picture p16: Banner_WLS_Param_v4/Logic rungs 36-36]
   36: XIC(Local_Control.5)XIO(Local_Control.6)GEQ(WLS.Command,19)LEQ(WLS.Command,22)BTD(Port_Data.Data_Transfer[0],0,WLS.Write.LM_Config.LT_Config[IndexR].Light_Control.Direction,0,8)BTD(Port_Data.Data_Transfer[1],0,WLS.Write.LM_Config.LT_Config[IndexR].Light_Control.Percent_Width_C1,0,8)BTD(Port_Data.Data_Transfer[2],0,WLS.Write.LM_Config.LT_Config[IndexR].Light_Control.ScrollBounce,0,8)BTD(Port_Data.Data_Transfer[3],0,WLS.Write.LM_Config.LT_Config[IndexR].Light_Control.Color_2_Intensity,0,8)BTD(Port_Data.Data_Transfer[4],0,WLS.Write.LM_Config.LT_Config[IndexR].Light_Control.Color_2,0,8)BTD(Port_Data.Data_Transfer[5],0,WLS.Write.LM_Config.LT_Config[IndexR].Light_Control.Pulse_Pattern,0,8)BTD(Port_Data.Data_Transfer[6],0,WLS.Write.LM_Config.LT_Config[IndexR].Light_Control.Speed,0,8)BTD(Port_Data.Data_Transfer[7],0,WLS.Write.LM_Config.LT_Config[IndexR].Light_Control.Color_1_Intensity,0,8)BTD(Port_Data.Data_Transfer[8],0,WLS.Write.LM_Config.LT_Config[IndexR].Light_Control.Color_1,0,8)BTD(Port_Data.Data_Transfer[9],0,WLS.Write.LM_Config.LT_Config[IndexR].Light_Control.Animation,0,8)BTD(Port_Data.Data_Transfer[10],0,WLS.Write.LM_Config.LT_Config[IndexR].Threshold_Override,0,8)BTD(Port_Data.Data_Transfer[11],0,WLS.Write.LM_Config.LT_Config[IndexR].Threshold_Comparison,0,8)BTD(Port_Data.Data_Transfer[12],0,WLS.Write.LM_Config.LT_Config[IndexR].Threshold_Value,0,8)BTD(Port_Data.Data_Transfer[13],0,WLS.Write.LM_Config.LT_Config[IndexR].Threshold_Enable,0,8)OTU(Port_Data.Port_Read.[Port])OTL(Local_Control.6);
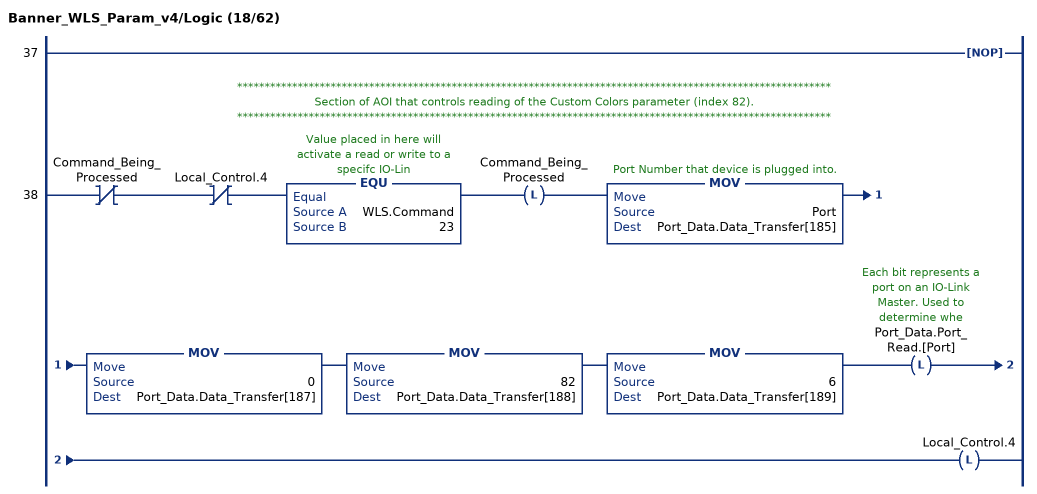
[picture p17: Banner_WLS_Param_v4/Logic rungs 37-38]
   37: NOP();
   // ************************************************************************************************************
   // Section of AOI that controls reading of the Custom Colors parameter (index 82).
   // ************************************************************************************************************
   38: XIO(Command_Being_Processed)XIO(Local_Control.4)EQU(WLS.Command,23)OTL(Command_Being_Processed)MOV(Port,Port_Data.Data_Transfer[185])MOV(0,Port_Data.Data_Transfer[187])MOV(82,Port_Data.Data_Transfer[188])MOV(6,Port_Data.Data_Transfer[189])OTL(Port_Data.Port_Read.[Port])OTL(Local_Control.4);
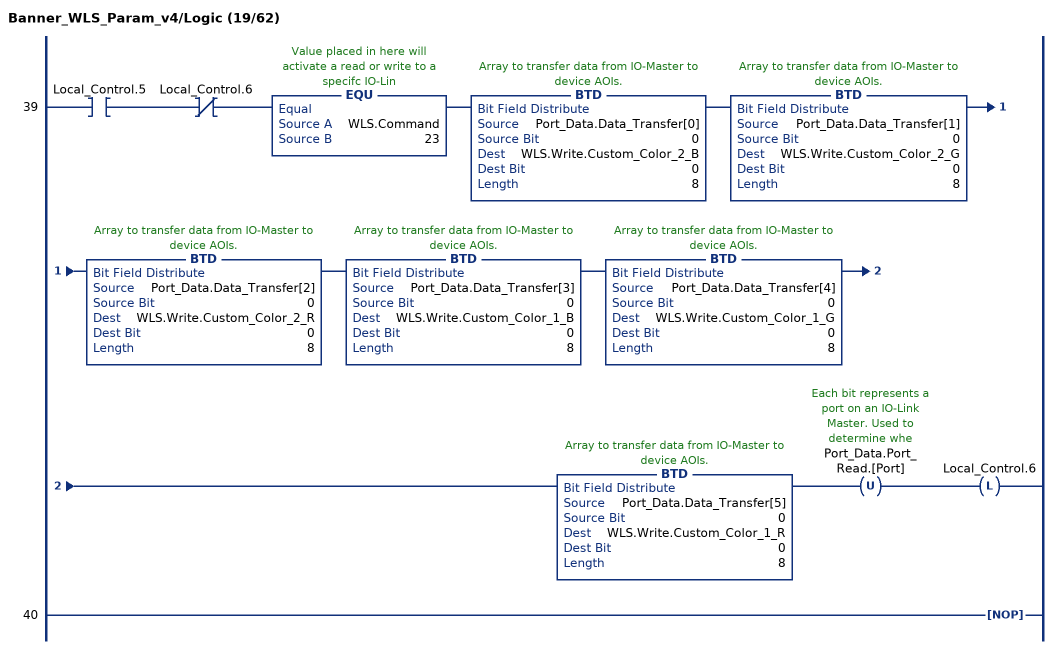
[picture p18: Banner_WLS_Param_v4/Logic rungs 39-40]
   39: XIC(Local_Control.5)XIO(Local_Control.6)EQU(WLS.Command,23)BTD(Port_Data.Data_Transfer[0],0,WLS.Write.Custom_Color_2_B,0,8)BTD(Port_Data.Data_Transfer[1],0,WLS.Write.Custom_Color_2_G,0,8)BTD(Port_Data.Data_Transfer[2],0,WLS.Write.Custom_Color_2_R,0,8)BTD(Port_Data.Data_Transfer[3],0,WLS.Write.Custom_Color_1_B,0,8)BTD(Port_Data.Data_Transfer[4],0,WLS.Write.Custom_Color_1_G,0,8)BTD(Port_Data.Data_Transfer[5],0,WLS.Write.Custom_Color_1_R,0,8)OTU(Port_Data.Port_Read.[Port])OTL(Local_Control.6);
   40: NOP();
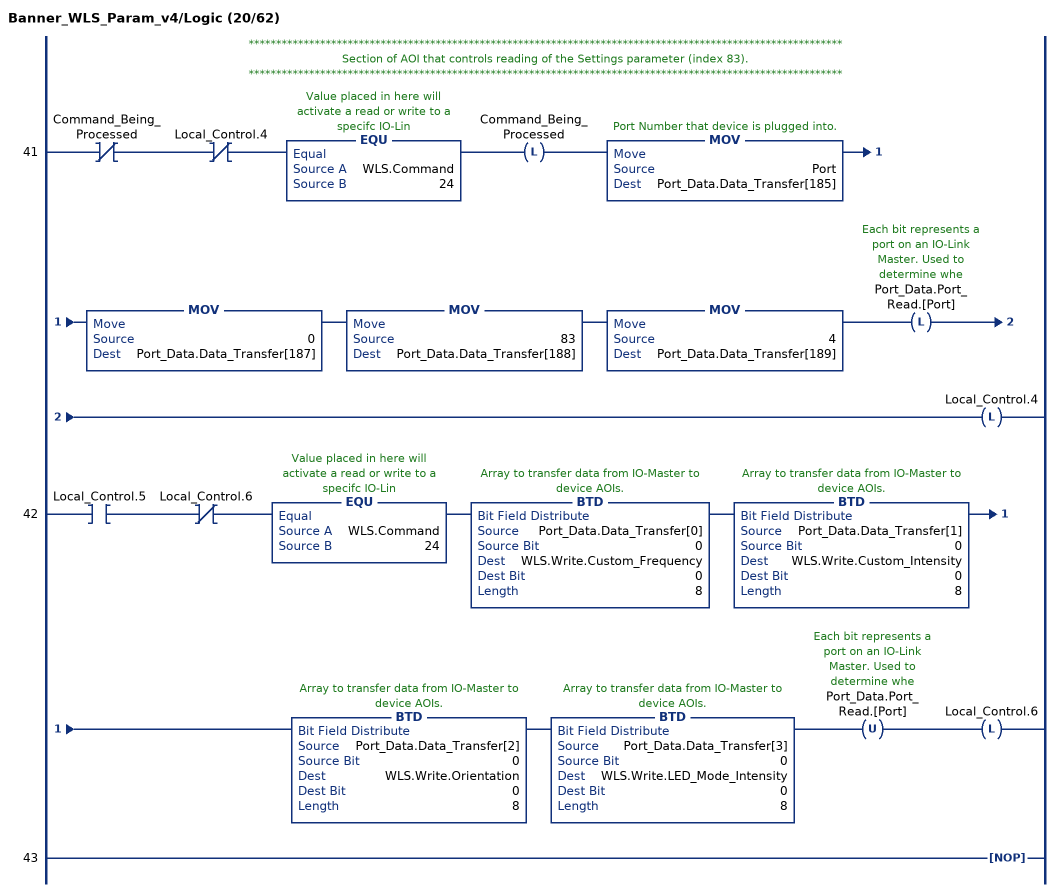
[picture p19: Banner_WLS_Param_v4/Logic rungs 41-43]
   // ************************************************************************************************************
   // Section of AOI that controls reading of the Settings parameter (index 83).
   // ************************************************************************************************************
   41: XIO(Command_Being_Processed)XIO(Local_Control.4)EQU(WLS.Command,24)OTL(Command_Being_Processed)MOV(Port,Port_Data.Data_Transfer[185])MOV(0,Port_Data.Data_Transfer[187])MOV(83,Port_Data.Data_Transfer[188])MOV(4,Port_Data.Data_Transfer[189])OTL(Port_Data.Port_Read.[Port])OTL(Local_Control.4);
   42: XIC(Local_Control.5)XIO(Local_Control.6)EQU(WLS.Command,24)BTD(Port_Data.Data_Transfer[0],0,WLS.Write.Custom_Frequency,0,8)BTD(Port_Data.Data_Transfer[1],0,WLS.Write.Custom_Intensity,0,8)BTD(Port_Data.Data_Transfer[2],0,WLS.Write.Orientation,0,8)BTD(Port_Data.Data_Transfer[3],0,WLS.Write.LED_Mode_Intensity,0,8)OTU(Port_Data.Port_Read.[Port])OTL(Local_Control.6);
   43: NOP();
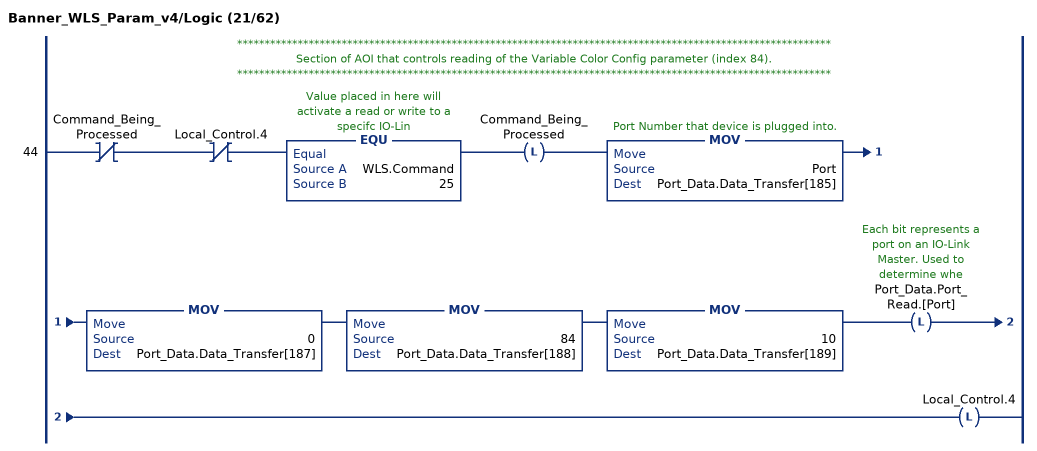
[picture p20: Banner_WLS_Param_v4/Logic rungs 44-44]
   // ************************************************************************************************************
   // Section of AOI that controls reading of the Variable Color Config parameter (index 84).
   // ************************************************************************************************************
   44: XIO(Command_Being_Processed)XIO(Local_Control.4)EQU(WLS.Command,25)OTL(Command_Being_Processed)MOV(Port,Port_Data.Data_Transfer[185])MOV(0,Port_Data.Data_Transfer[187])MOV(84,Port_Data.Data_Transfer[188])MOV(10,Port_Data.Data_Transfer[189])OTL(Port_Data.Port_Read.[Port])OTL(Local_Control.4);
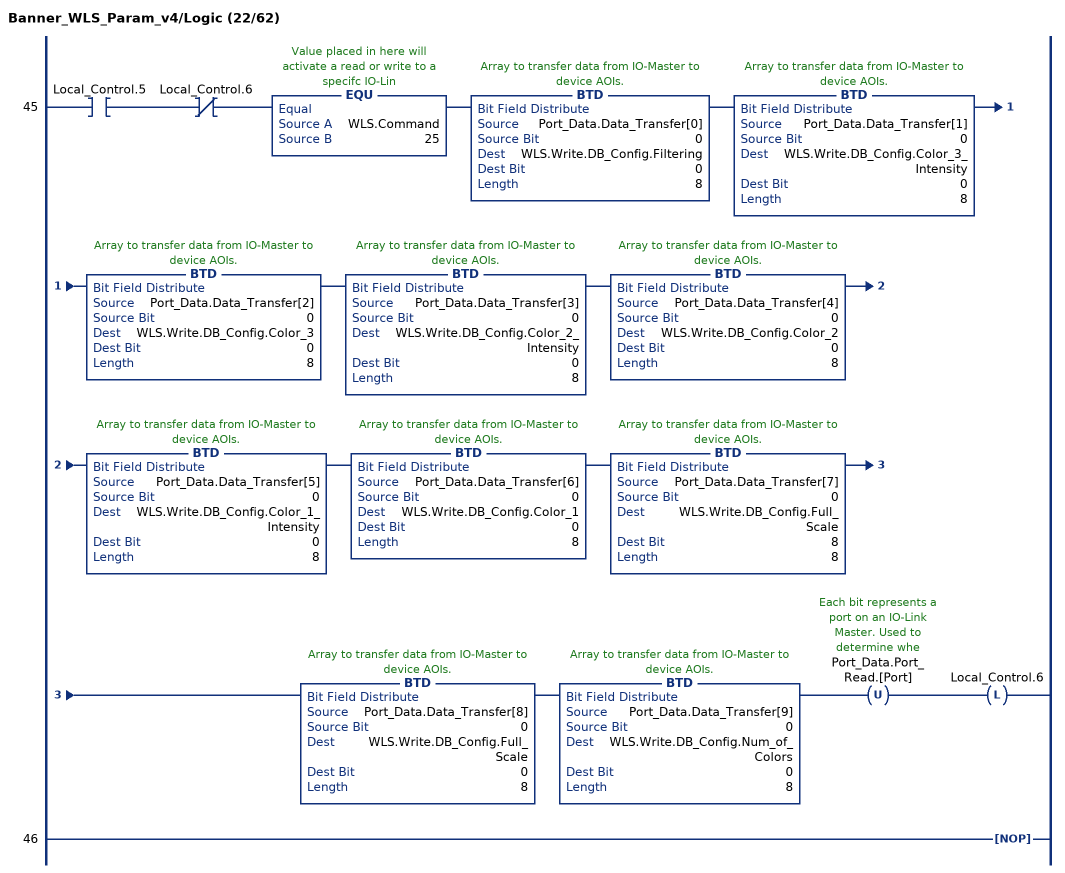
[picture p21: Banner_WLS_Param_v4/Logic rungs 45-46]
   45: XIC(Local_Control.5)XIO(Local_Control.6)EQU(WLS.Command,25)BTD(Port_Data.Data_Transfer[0],0,WLS.Write.DB_Config.Filtering,0,8)BTD(Port_Data.Data_Transfer[1],0,WLS.Write.DB_Config.Color_3_Intensity,0,8)BTD(Port_Data.Data_Transfer[2],0,WLS.Write.DB_Config.Color_3,0,8)BTD(Port_Data.Data_Transfer[3],0,WLS.Write.DB_Config.Color_2_Intensity,0,8)BTD(Port_Data.Data_Transfer[4],0,WLS.Write.DB_Config.Color_2,0,8)BTD(Port_Data.Data_Transfer[5],0,WLS.Write.DB_Config.Color_1_Intensity,0,8)BTD(Port_Data.Data_Transfer[6],0,WLS.Write.DB_Config.Color_1,0,8)BTD(Port_Data.Data_Transfer[7],0,WLS.Write.DB_Config.Full_Scale,8,8)BTD(Port_Data.Data_Transfer[8],0,WLS.Write.DB_Config.Full_Scale,0,8)BTD(Port_Data.Data_Transfer[9],0,WLS.Write.DB_Config.Num_of_Colors,0,8)OTU(Port_Data.Port_Read.[Port])OTL(Local_Control.6);
   46: NOP();
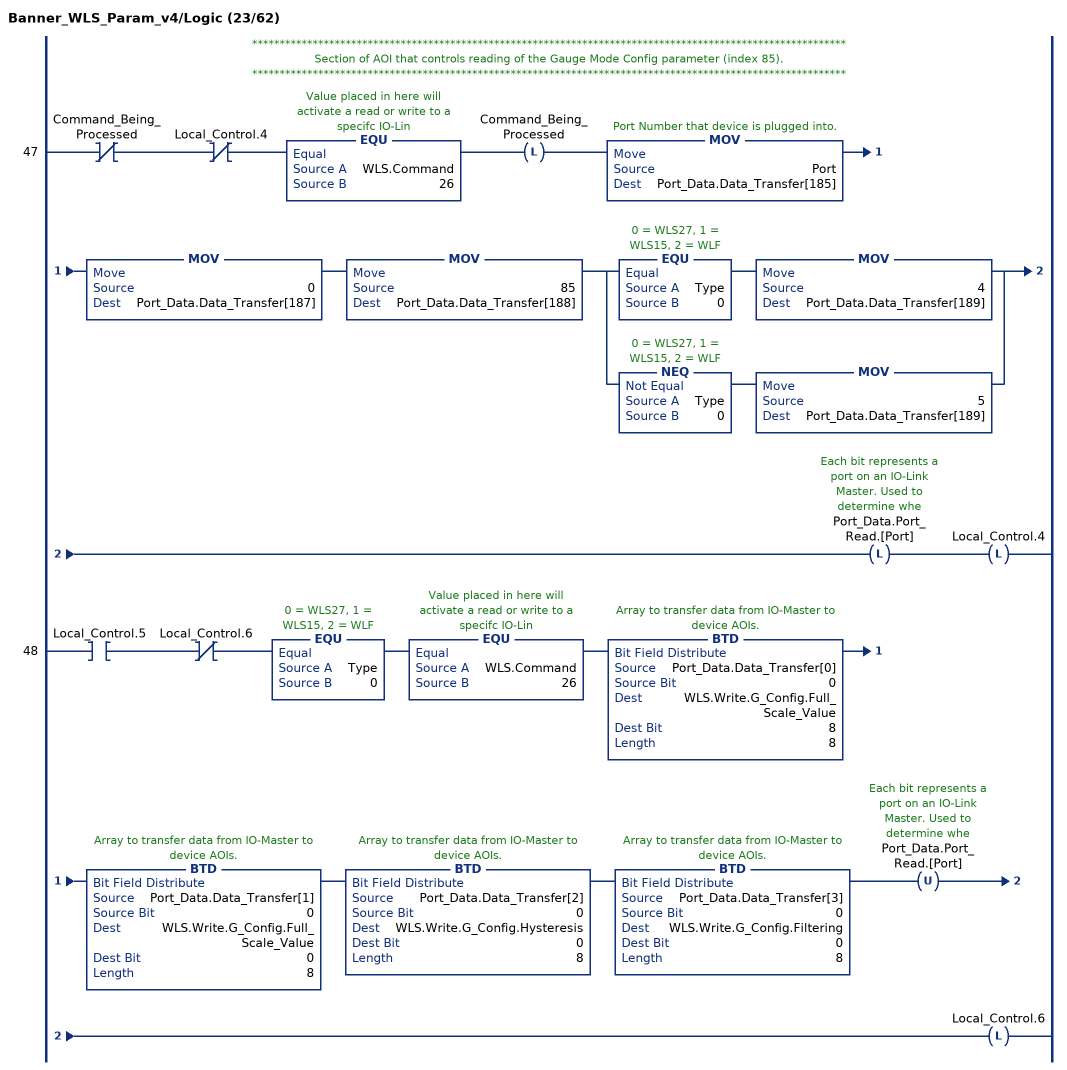
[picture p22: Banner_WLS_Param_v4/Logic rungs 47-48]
   // ************************************************************************************************************
   // Section of AOI that controls reading of the Gauge Mode Config parameter (index 85).
   // ************************************************************************************************************
   47: XIO(Command_Being_Processed)XIO(Local_Control.4)EQU(WLS.Command,26)OTL(Command_Being_Processed)MOV(Port,Port_Data.Data_Transfer[185])MOV(0,Port_Data.Data_Transfer[187])MOV(85,Port_Data.Data_Transfer[188])[EQU(Type,0) MOV(4,Port_Data.Data_Transfer[189]) ,NEQ(Type,0) MOV(5,Port_Data.Data_Transfer[189]) ]OTL(Port_Data.Port_Read.[Port])OTL(Local_Control.4);
   48: XIC(Local_Control.5)XIO(Local_Control.6)EQU(Type,0)EQU(WLS.Command,26)BTD(Port_Data.Data_Transfer[0],0,WLS.Write.G_Config.Full_Scale_Value,8,8)BTD(Port_Data.Data_Transfer[1],0,WLS.Write.G_Config.Full_Scale_Value,0,8)BTD(Port_Data.Data_Transfer[2],0,WLS.Write.G_Config.Hysteresis,0,8)BTD(Port_Data.Data_Transfer[3],0,WLS.Write.G_Config.Filtering,0,8)OTU(Port_Data.Port_Read.[Port])OTL(Local_Control.6);
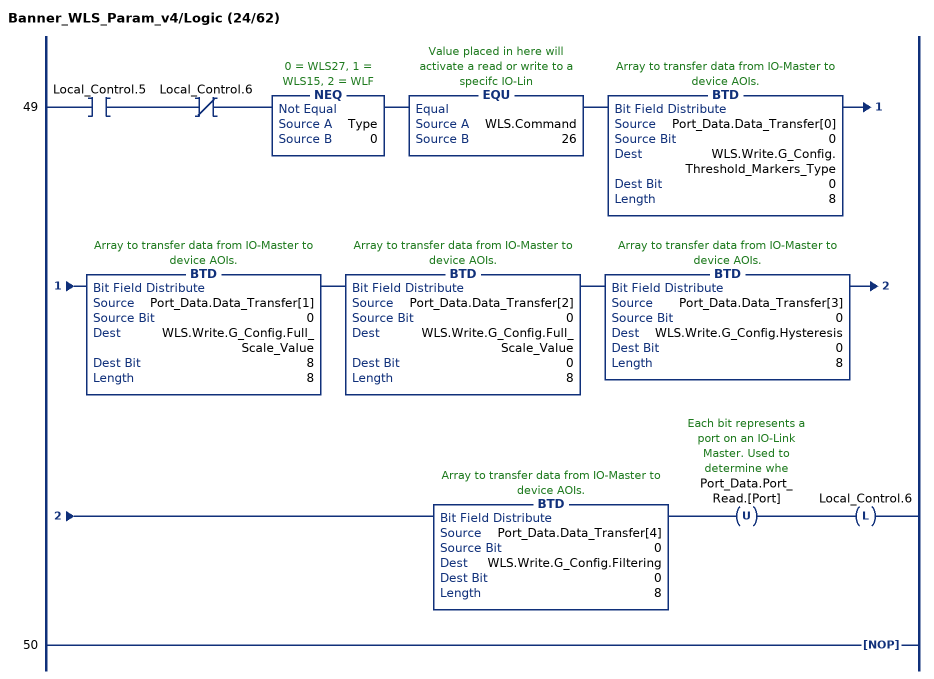
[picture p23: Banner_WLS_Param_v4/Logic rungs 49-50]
   49: XIC(Local_Control.5)XIO(Local_Control.6)NEQ(Type,0)EQU(WLS.Command,26)BTD(Port_Data.Data_Transfer[0],0,WLS.Write.G_Config.Threshold_Markers_Type,0,8)BTD(Port_Data.Data_Transfer[1],0,WLS.Write.G_Config.Full_Scale_Value,8,8)BTD(Port_Data.Data_Transfer[2],0,WLS.Write.G_Config.Full_Scale_Value,0,8)BTD(Port_Data.Data_Transfer[3],0,WLS.Write.G_Config.Hysteresis,0,8)BTD(Port_Data.Data_Transfer[4],0,WLS.Write.G_Config.Filtering,0,8)OTU(Port_Data.Port_Read.[Port])OTL(Local_Control.6);
   50: NOP();
